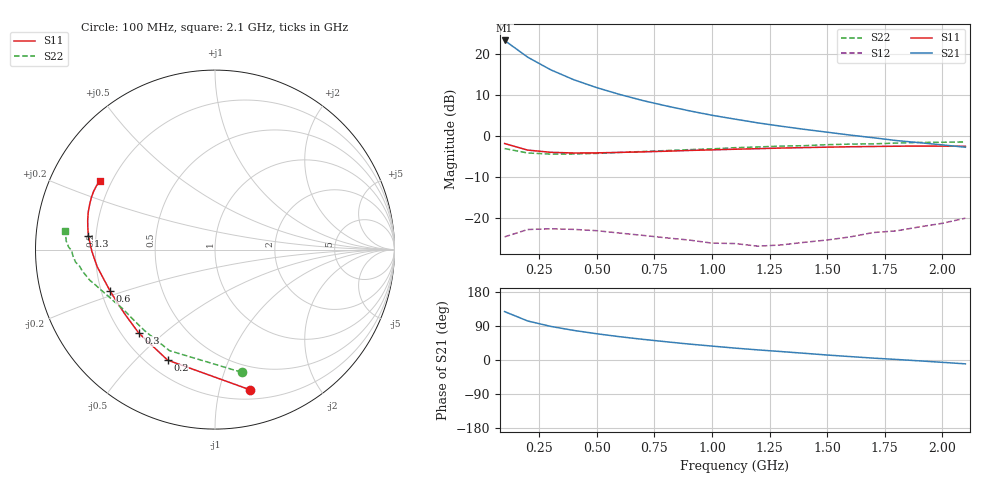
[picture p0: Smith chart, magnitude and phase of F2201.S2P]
! Date: Tue Aug 08 14:25:37 1995
# MHZ  S  MA  R  50.0000
!  POLYFET RF DEVICES
!  F2201
!  S PARAMETERS
!  VDS=12.5V, IDQ=200mA
!FREQ  S11MAG S11ANG S21MAG S21ANG S12MAG S12ANG S22MAG S22ANG
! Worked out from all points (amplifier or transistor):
!   21 points, 100 MHz to 2.1 GHz, reference 50 ohm
!   highest |S21| = 23.3 dB at 100 MHz (marker M1)
!   |S21| within 3 dB of that: start of sweep to 173.5 MHz
!   unconditionally stable (mu >= 1): 893.6 MHz to 1.702 GHz
!   at 400 MHz: K = 0.37, MSG = 18.3 dB, |S12| = -22.9 dB
!   at 1.1 GHz: K = 1.24, MAG = 12.3 dB, |S12| = -26.3 dB
!   at 2.1 GHz: K = 0.60, MSG = 8.7 dB, |S12| = -20.1 dB
!   S11 on the Smith chart (normalised r, x): 100 MHz: 0.28, -1.24; 200 MHz: 0.28, -0.62; 300 MHz: 0.27, -0.41; 600 MHz: 0.24, -0.18; 1.3 GHz: 0.17, +0.05; 2.1 GHz: 0.16, +0.27
100  0.8062 -75.9  14.66 127.7  0.05825 40.9  0.6993 -77.8
200  0.67 -113.2  9.165 103.0  0.07163 20.2  0.6176 -114.2
300  0.6296 -132.5  6.422 88.7  0.07307 9.4  0.5984 -131.3
400  0.6175 -144.2  4.858 78.1  0.07192 3.3  0.6008 -141.0
500  0.6196 -152.2  3.884 69.3  0.06931 -1.5  0.6105 -147.3
600  0.6281 -158.3  3.206 61.4  0.06479 -4.4  0.6273 -151.6
700  0.6374 -163.5  2.702 54.5  0.06076 -6.0  0.6442 -155.5
800  0.6489 -167.8  2.328 48.2  0.05672 -5.8  0.6609 -158.5
900  0.6633 -171.8  2.029 42.1  0.0533 -4.6  0.6783 -161.2
1000  0.6742 -175.7  1.785 36.7  0.04885 -1.7  0.6937 -163.4
1100  0.6865 -179.3  1.601 31.4  0.04826 3.3  0.7172 -166.1
1200  0.6974 177.1  1.44 26.7  0.04483 10.0  0.732 -168.4
1300  0.7096 173.7  1.313 22.3  0.04641 17.7  0.7497 -171.0
1400  0.7187 170.3  1.203 17.8  0.04994 24.3  0.7587 -172.8
1500  0.7276 167.1  1.109 13.1  0.05334 27.5  0.7803 -174.9
1600  0.736 163.8  1.022 9.0  0.05821 30.8  0.7925 -177.6
1700  0.7416 160.6  0.9488 5.0  0.06579 31.7  0.7989 -179.6
1800  0.7472 157.4  0.8767 1.5  0.06894 32.7  0.8158 179.0
1900  0.7502 154.4  0.8257 -2.2  0.07707 34.4  0.8306 176.6
2000  0.7499 151.7  0.7752 -6.2  0.08533 33.8  0.8358 174.3
2100  0.7452 149.1  0.726 -10.2  0.09855 30.2  0.8425 172.9
